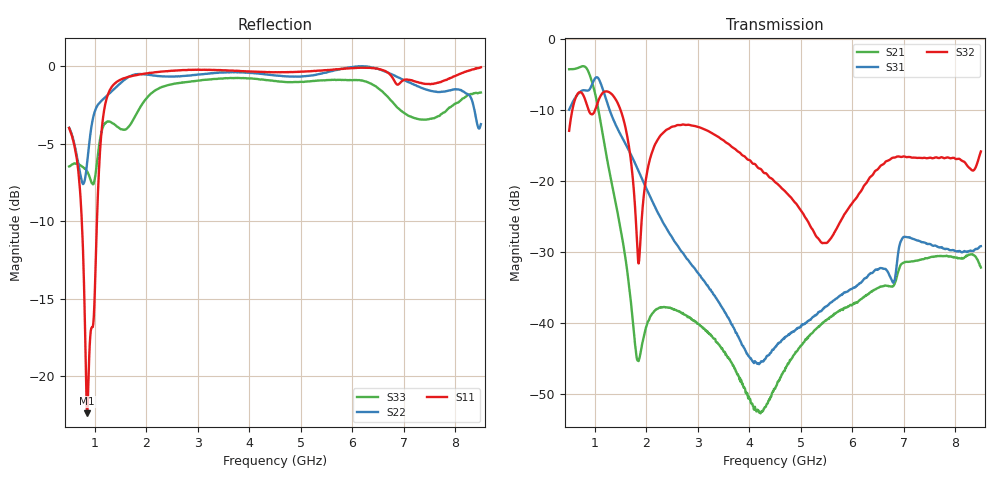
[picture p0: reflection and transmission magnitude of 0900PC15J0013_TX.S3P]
! Pin3 (TRX) is connected to port3, port impedance: 0.1ohms
! Pin4 (PA) is connected to port2, port impedance: 40-j49
! Pin7 (ANT) is connected to port1. port impedance: 50ohms
!PINS 1/2 (LNA_N/LNA_P) are terminated with 50ohm load.
# Hz S RI R 50
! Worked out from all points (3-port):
!   801 points, 500 MHz to 8.5 GHz, reference 50 ohm
!   strongest paths, dB at 500 MHz, 2.5 GHz, 4.5 GHz, 6.5 GHz, 8.5 GHz:
!     S32: -13.0, -12.4, -20.2, -18.4, -15.9
!     S31: -10.0, -28.0, -43.5, -32.5, -29.2
!     S21: -4.3, -38.0, -49.3, -35.1, -32.2
!   lowest |S11| = -22.4 dB at 850 MHz (marker M1), VSWR 1.16, Z = 54.7 - j6.45 ohm
!   |S11| at or under -10 dB: 746.6 MHz to 1.041 GHz (294 MHz wide, 32.9 % of centre)
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5e8  0.3858 -0.5005  0.0855 -0.6038  0.2922 0.1287
     0.0853 -0.6038  0.0954 0.6252  0.1112 0.1973
     0.29 0.1269  0.1104 0.1956  0.1908 -0.4348
8.5e8  0.0482 -0.0587  -0.5882 0.1612  0.0272 -0.4284
       -0.5883 0.1613  0.2581 0.4142  0.3362 -0.0144
       0.0315 -0.4296  0.3382 -0.011  -0.4464 -0.101
1.1e9  0.4944 0.1908  0.083 0.2601  -0.4859 -0.0947
       0.0829 0.2602  0.6568 0.3902  0.385 0.00795
       -0.4894 -0.1001  0.3884 0.0116  -0.5733 0.0822
1.44e9  0.6291 -0.6335  0.0596 0.00597  -0.0711 0.2211
        0.0597 0.00598  0.8627 0.0215  0.2351 -0.2643
        -0.0686 0.2225  0.2323 -0.2678  0.0205 0.6369
1.83e9  0.1302 -0.9283  0.00514 0.00134  0.0954 0.0747
        0.00525 0.00134  0.8095 -0.4822  0.0158 -0.0267
        0.094 0.0765  0.0163 -0.0264  0.6087 -0.37
2.49e9  -0.4223 -0.869  0.0114 0.0053  0.0373 -0.0125
        0.0115 0.00539  0.3224 -0.8672  0.2328 -0.00485
        0.0384 -0.0129  0.2392 -0.00582  -0.3463 -0.8011
4.5e9  -0.9552 -0.0338  0.0017 0.00303  0.0064 0.00251
       0.00167 0.00298  -0.6518 -0.6682  0.063 -0.0778
       0.00618 0.00258  0.0628 -0.0751  -0.8899 0.1015
5.48e9  -0.8961 0.3731  0.0044 0.00923  0.0102 0.00756
        0.00441 0.00939  -0.9482 -0.0894  0.0355 -0.00465
        0.0106 0.00751  0.036 -0.00585  -0.8214 0.3669
6.52e9  -0.8328 0.513  0.0105 0.0141  0.0213 0.0105
        0.0107 0.0141  -0.9772 -0.000566  0.0871 0.0858
        0.021 0.0114  0.0842 0.0899  -0.6614 0.5253
8.5e9  -0.013 0.9912  0.0234 -0.00707  0.0343 -0.00679
       0.0234 -0.00722  -0.2218 0.6108  0.1482 0.062
       0.0338 -0.00749  0.1496 0.0586  -0.1026 0.8153
